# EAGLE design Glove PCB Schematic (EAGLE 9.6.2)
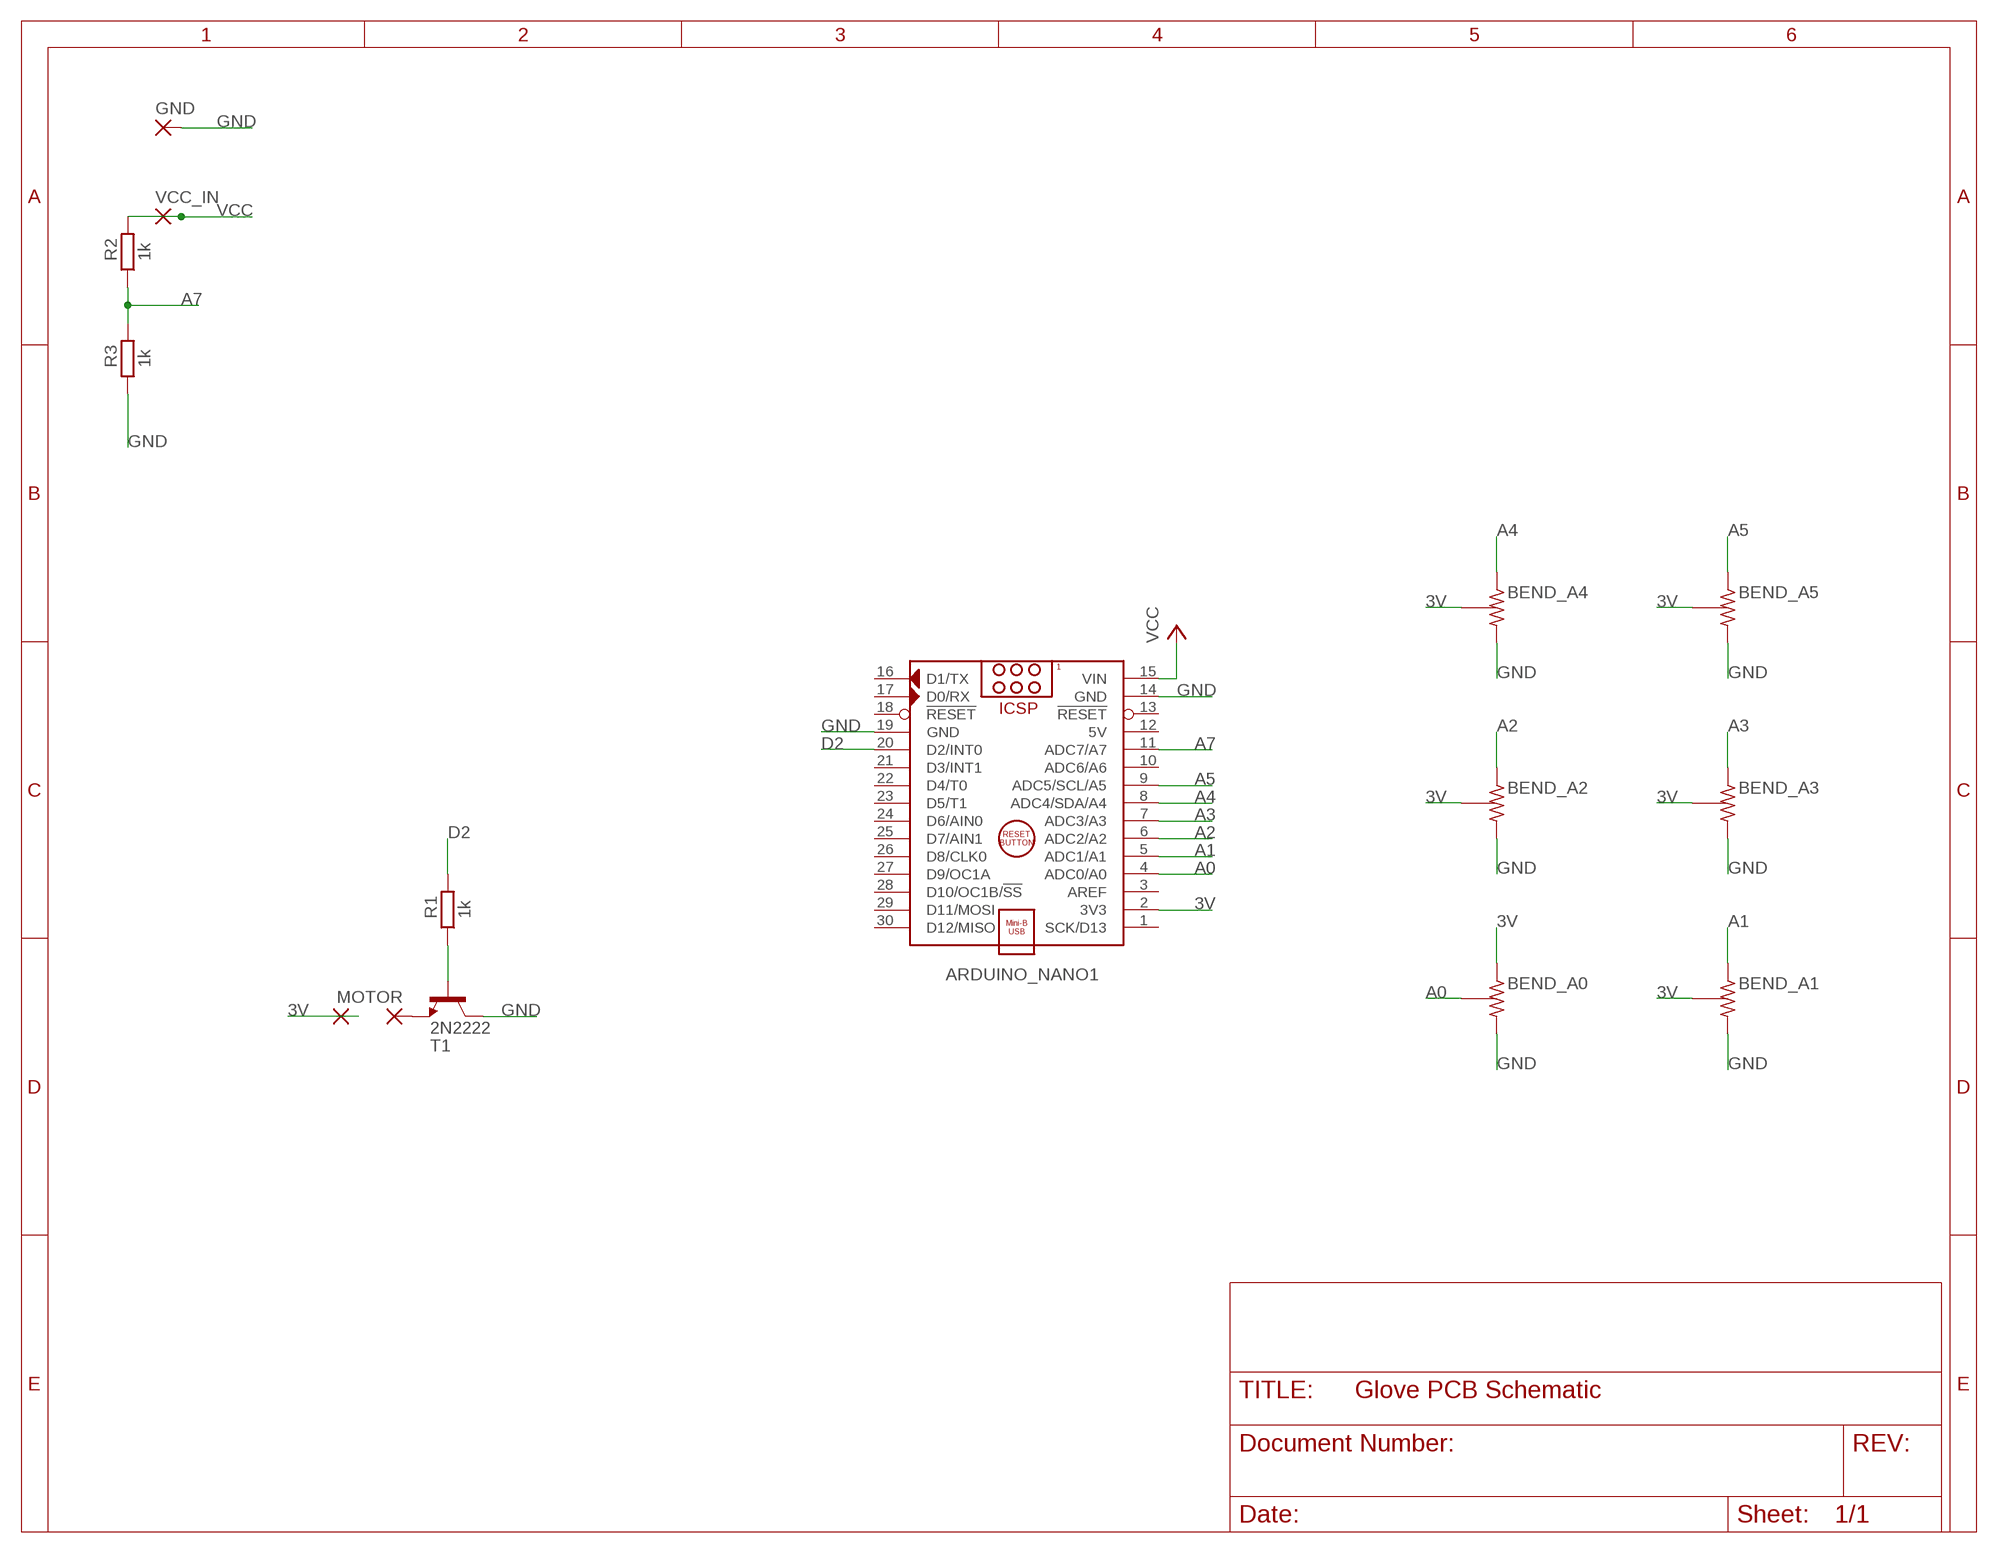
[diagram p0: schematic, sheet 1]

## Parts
ARDUINO_NANO1  ARDUINO_NANO  [ARDUINO_NANO]
BEND_A0  BEND_SENSOR  [BEND_SENSOR]
BEND_A1  BEND_SENSOR  [BEND_SENSOR]
BEND_A2  BEND_SENSOR  [BEND_SENSOR]
BEND_A3  BEND_SENSOR  [BEND_SENSOR]
BEND_A4  BEND_SENSOR  [BEND_SENSOR]
BEND_A5  BEND_SENSOR  [BEND_SENSOR]
GND  WIREPAD1,6/0,9  [1,6/0,9]
GND1  WIREPAD1,6/0,9  [1,6/0,9]
MOTOR  WIREPAD1,6/0,9  [1,6/0,9]
R1  1k  R-EU_0204/7  [0204/7]
R2  1k  R-EU_0204/7  [0204/7]
R3  1k  R-EU_0204/7  [0204/7]
T1  2N2222  [TO18]
VCC_IN  WIREPAD1,6/0,9  [1,6/0,9]

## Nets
3V: ARDUINO_NANO1.2(3V3) BEND_A0.P$1 BEND_A1.P$3 BEND_A2.P$3 BEND_A3.P$3 BEND_A4.P$3 BEND_A5.P$3 MOTOR.1(P)
A0: ARDUINO_NANO1.4(ADC0/A0) BEND_A0.P$3
A1: ARDUINO_NANO1.5(ADC1/A1) BEND_A1.P$1
A2: ARDUINO_NANO1.6(ADC2/A2) BEND_A2.P$1
A3: ARDUINO_NANO1.7(ADC3/A3) BEND_A3.P$1
A4: ARDUINO_NANO1.8(ADC4/SDA/A4) BEND_A4.P$1
A5: ARDUINO_NANO1.9(ADC5/SCL/A5) BEND_A5.P$1
A7: ARDUINO_NANO1.11(ADC7/A7) R2.1 R3.2
D2: ARDUINO_NANO1.20(D2/INT0) R1.2
GND: ARDUINO_NANO1.14(GND) ARDUINO_NANO1.19(GND) BEND_A0.P$2 BEND_A1.P$2 BEND_A2.P$2 BEND_A3.P$2 BEND_A4.P$2 BEND_A5.P$2 GND.1(P) R3.1 T1.3(C)
N$1: R1.1 T1.2(B)
N$2: GND1.1(P) T1.1(E)
VCC: ARDUINO_NANO1.15(VIN) R2.2 VCC_IN.1(P)
Unconnected: ARDUINO_NANO1.1(SCK/D13) ARDUINO_NANO1.3(AREF) ARDUINO_NANO1.10(ADC6/A6) ARDUINO_NANO1.13(!RESET) ARDUINO_NANO1.16(D1/TX) ARDUINO_NANO1.17(D0/RX) ARDUINO_NANO1.18(!RESET) ARDUINO_NANO1.21(D3/INT1) ARDUINO_NANO1.22(D4/T0) ARDUINO_NANO1.23(D5/T1) ARDUINO_NANO1.24(D6/AIN0) ARDUINO_NANO1.25(D7/AIN1) ARDUINO_NANO1.26(D8/CLK0) ARDUINO_NANO1.27(D9/OC1A) ARDUINO_NANO1.28(D10/OC1B/!SS) ARDUINO_NANO1.29(D11/MOSI) ARDUINO_NANO1.30(D12/MISO)

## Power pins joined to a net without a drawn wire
5V: ARDUINO_NANO1.12(5V)

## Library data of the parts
ARDUINO_NANO1 = ArduinoNanoV30:ARDUINO_NANO: Arduino Nano V3.0 Module Overview: The Arduino Nano is a small, complete, and breadboard-friendly board based on the ATmega328 (Arduino Nano 3.x) or ATmega168 (Arduino Nano 2.x). It has more or less the same functionality of the Arduino Duemilanove, but in a different package. It lacks only a DC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
BEND_A0 BEND_A1-BEND_A5 = Glove PCB:BEND_SENSOR
GND GND1 MOTOR VCC_IN = wirepad:WIREPAD: Wire PAD connect wire on PCB
R1-R3 = rcl:R-EU_: RESISTOR, European symbol; SPICEPREFIX: R
T1 = transistor:2N2222: NPN TRANSISTOR

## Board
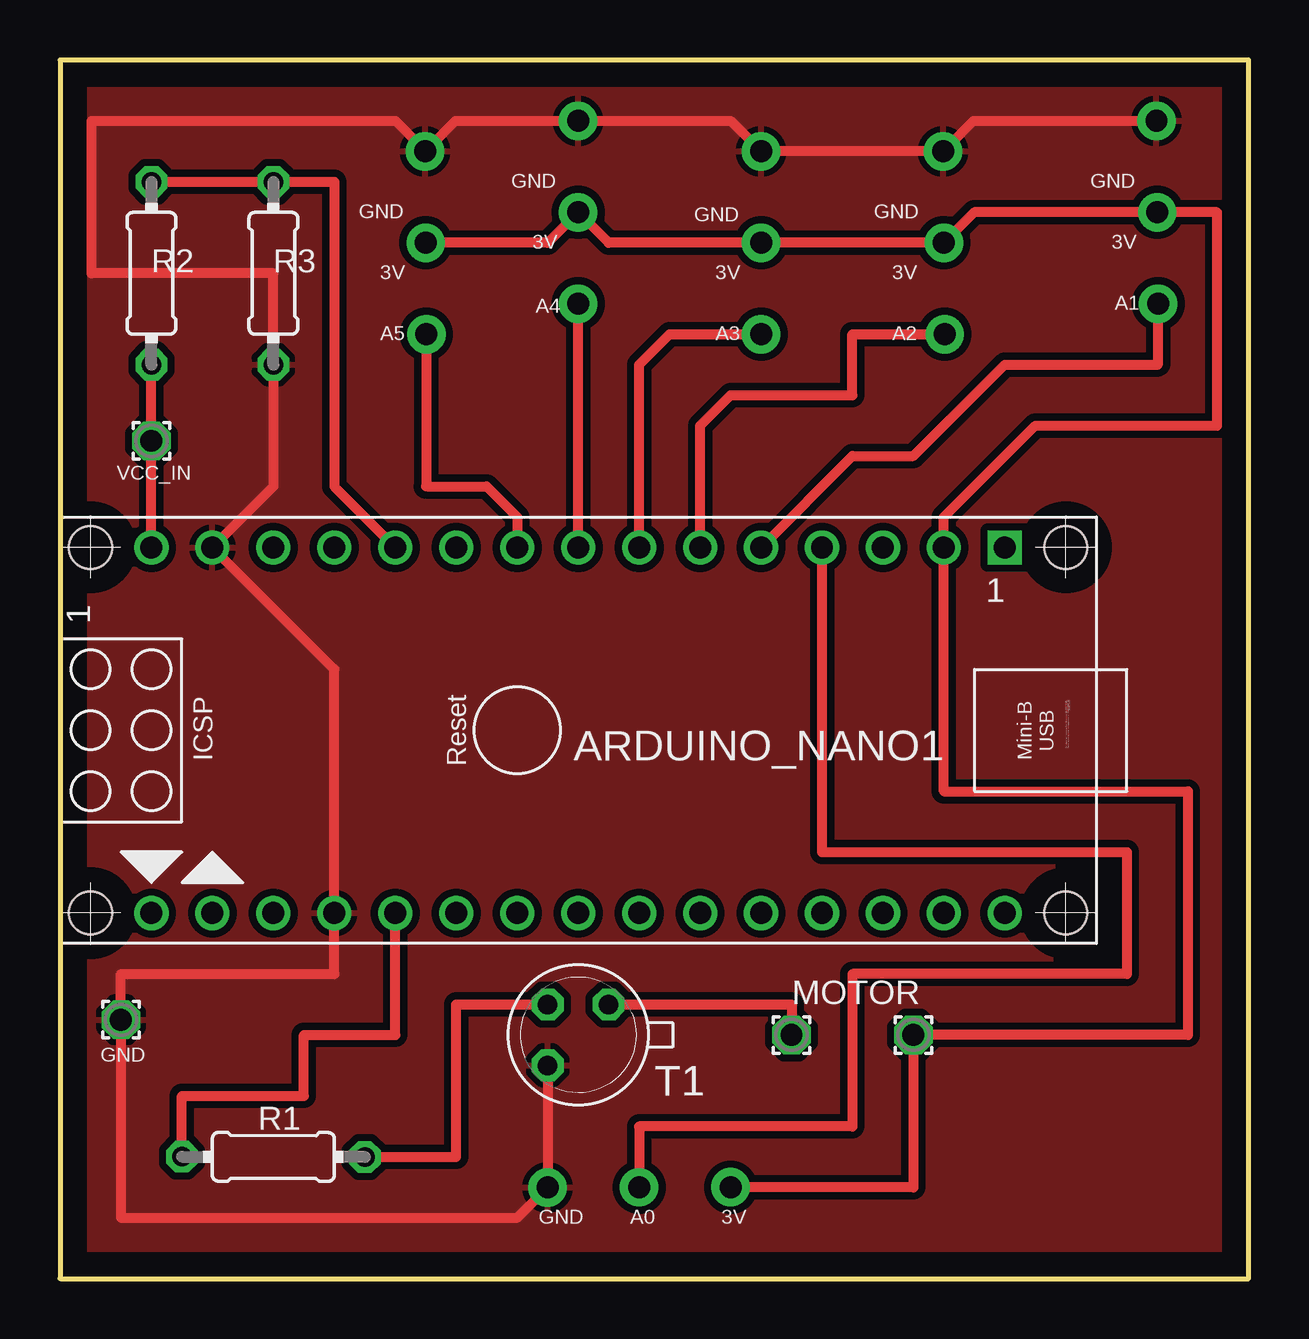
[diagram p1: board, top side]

Size 49.53 x 50.8 mm. Coordinates in mm from the lower left corner, seen from the top.
Outline: 0,0 49.53,0 49.53,50.8 0,50.8 0,0
Copper layers (1*16): Top 0.035mm / dielectric 1.5mm / Bottom 0.035mm
Design rules "default *": minimum track width 6mil, minimum drill 0.35mm, track to track 10mil, track to pad 35mil, pad to pad 6mil, via to via 6mil, smd to smd 6mil, copper to edge 40mil, drill to drill 6mil, minimum pad ring 10mil, minimum via ring 8mil, stop-mask expansion 4mil, vias tented up to drill 0mil, thermal gap 10mil

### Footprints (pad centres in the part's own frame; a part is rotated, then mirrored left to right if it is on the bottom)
ARDUINO_NANO = drill 0.914 square: 1 -20.32,-7.62 | drill 0.914: 2 -17.78,-7.62; 3 -15.24,-7.62; 4 -12.7,-7.62; 5 -10.16,-7.62; 6 -7.62,-7.62; 7 -5.08,-7.62; 8 -2.54,-7.62; 9 0,-7.62; 10 2.54,-7.62; 11 5.08,-7.62; 12 7.62,-7.62; 13 10.16,-7.62; 14 12.7,-7.62; 15 15.24,-7.62; 16 15.24,7.62; 17 12.7,7.62; 18 10.16,7.62; 19 7.62,7.62; 20 5.08,7.62; 21 2.54,7.62; 22 0,7.62; 23 -2.54,7.62; 24 -5.08,7.62; 25 -7.62,7.62; 26 -10.16,7.62; 27 -12.7,7.62; 28 -15.24,7.62; 29 -17.78,7.62; 30 -20.32,7.62 | hole 1.778: -22.86,-7.62; -22.86,7.62; 17.78,7.62; 17.78,-7.62
BEND_SENSOR = drill 0.914 pad 1.6: P$1 -3.81,0; P$2 3.81,0; P$3 0,0
1,6/0,9 = drill 0.914 pad 1.6 octagon: 1 0,0
0204/7 = drill 0.813 octagon: 1 -3.81,0; 2 3.81,0
TO18 = drill 0.813 octagon: 1 -1.27,-1.27; 2 1.27,-1.27; 3 1.27,1.27

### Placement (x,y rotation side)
ARDUINO_NANO1  19.05,22.86 180 top
BEND_A0  24.13,3.81 180.1 top
BEND_A1  45.72,44.45 90.5 top
BEND_A2  36.83,43.18 90.5 top
BEND_A3  29.21,43.18 90 top
BEND_A4  21.59,44.45 90 top
BEND_A5  15.24,43.18 90.4 top
GND  2.54,10.79 0 top
GND1  30.48,10.16 270 top
MOTOR  35.56,10.16 270 top
R1  8.89,5.08 179.9 top
R2  3.81,41.91 270 top
R3  8.89,41.91 90 top
T1  21.59,10.16 180 top
VCC_IN  3.81,34.92 0 top

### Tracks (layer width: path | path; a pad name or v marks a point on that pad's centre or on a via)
3V
  Top 0.406: BEND_A0.P$1 35.56,3.81 MOTOR.1 46.99,10.16 46.99,20.32 36.83,20.32 ARDUINO_NANO1.2 36.83,31.75 40.64,35.56 48.21,35.56 48.21,44.45 BEND_A1.P$3 38.1,44.45 BEND_A2.P$3 BEND_A3.P$3 22.86,43.18 BEND_A4.P$3 20.32,43.18 BEND_A5.P$3
A0
  Top 0.406: ARDUINO_NANO1.4 31.75,17.78 44.45,17.78 44.45,12.7 33.02,12.7 33.02,6.35 24.13,6.35 BEND_A0.P$3
A1
  Top 0.406: ARDUINO_NANO1.5 33.02,34.29 35.56,34.29 39.37,38.1 45.72,38.1 45.75,38.13 BEND_A1.P$1
A2
  Top 0.406: ARDUINO_NANO1.6 26.67,35.56 27.94,36.83 33.02,36.83 33.02,39.37 | 33.02,39.37 | 33.02,39.37 BEND_A2.P$1
A3
  Top 0.406: ARDUINO_NANO1.7 24.13,38.1 25.4,39.37 BEND_A3.P$1
A4
  Top 0.406: ARDUINO_NANO1.8 BEND_A4.P$1
A5
  Top 0.406: BEND_A5.P$1 15.27,33.05 | 15.27,33.05 15.24,33.02 | 15.27,33.05 15.29,33.02 17.78,33.02 19.05,31.75 ARDUINO_NANO1.9
A7
  Top 0.406: R2.1 R3.2 11.43,45.72 11.43,33.02 ARDUINO_NANO1.11
D2
  Top 0.406: ARDUINO_NANO1.20 13.97,10.16 10.16,10.16 10.16,7.62 5.08,7.62 R1.2 | R1.2
GND
  Top 0.406: T1.3 BEND_A0.P$2 19.06,2.54 2.54,2.54 GND.1 2.54,12.7 11.43,12.7 ARDUINO_NANO1.19 11.43,25.4 ARDUINO_NANO1.14 8.89,33.02 R3.1 8.89,41.91 1.32,41.91 1.32,48.26 13.97,48.26 15.21,47.02 BEND_A5.P$2 16.48,48.26 BEND_A4.P$2 27.94,48.26 BEND_A3.P$2 BEND_A2.P$2 | BEND_A2.P$2 | BEND_A2.P$2 38.07,48.26 BEND_A1.P$2
  pour Top (isolate 0.305): 0,0 49.53,0 49.53,50.8 0,50.8
N$1
  Top 0.406: R1.1 16.51,5.08 16.51,11.43 T1.2
N$2
  Top 0.406: T1.1 30.48,11.43 GND1.1
VCC
  Top 0.406: ARDUINO_NANO1.15 VCC_IN.1 R2.2

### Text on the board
tPlace: GND | GND | GND | GND | GND | 3V | 3V | 3V | 3V | 3V | A4 | A1 | A5 | A3 | A2 | GND | A0 | 3V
